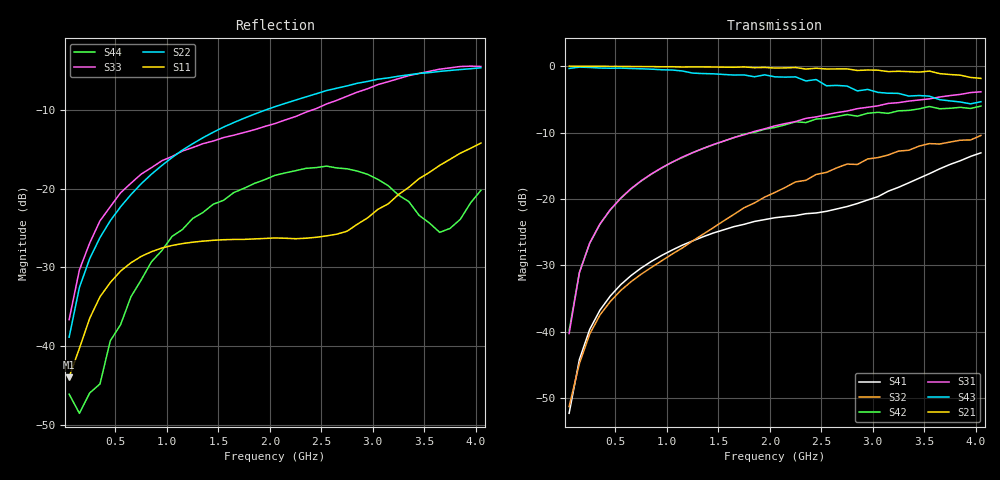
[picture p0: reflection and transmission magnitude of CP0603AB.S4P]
! Network Analyzer HP8720D.07.14 Serial No. US38111185
! 28 Apr 1999  02:06:29
! Frequency 	S11		S21		S31		S41		S12		S22		S23		S24		S13		S23		S33		S34		S14		S24		S34		S44
# HZ  S  DB R 50
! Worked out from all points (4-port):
!   41 points, 50 MHz to 4.05 GHz, reference 50 ohm
!   strongest paths, dB at 50 MHz, 1.05 GHz, 2.05 GHz, 3.05 GHz, 4.05 GHz:
!     S21: 0.0, -0.1, -0.3, -0.6, -1.9
!     S43: -0.4, -0.6, -1.6, -4.0, -5.4
!     S31: -40.2, -14.5, -9.0, -6.0, -3.9
!     S42: -39.8, -14.5, -9.2, -7.0, -6.0
!     S32: -51.2, -28.3, -19.0, -13.8, -10.4
!     S41: -52.2, -27.7, -22.8, -19.6, -13.1
!   lowest |S11| = -43.9 dB at 50 MHz (marker M1), VSWR 1.01, Z = 50.6 - j0.257 ohm
!   |S11| at or under -10 dB: start of sweep to end of sweep
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5e7  -43.93 -23.6  -0.01 -1.1  -41.46 90.6  -52.89 115.5
     -0.02 -0.7  -38.86 41.2  -51.21 84.4  -40.47 85.8
     -40.25 86.7  -51.23 88.0  -36.63 43.5  -0.06 -2.0
     -52.25 97.0  -39.79 80.3  -0.36 -1.7  -46.09 -17.5
1.5e8  -40.27 -64.9  -0.03 -2.4  -31.01 85.8  -44.19 88.0
       -0.03 -2.4  -32.53 55.9  -44.90 88.9  -31.02 85.7
       -31.08 85.5  -44.76 87.7  -30.31 65.5  -0.07 -5.1
       -44.15 87.9  -31.05 85.6  -0.16 -5.0  -48.53 -14.9
2.5e8  -36.46 -80.7  -0.02 -4.0  -26.62 83.1  -39.63 85.8
       -0.04 -4.0  -28.88 59.3  -40.24 86.7  -26.68 82.7
       -26.63 83.2  -40.32 86.8  -26.89 66.4  -0.10 -8.4
       -39.62 85.6  -26.67 82.3  -0.21 -8.3  -45.95 -77.3
9.5e8  -27.53 -129.4  -0.10 -14.9  -15.25 66.3  -28.43 74.9
       -0.11 -15.0  -17.04 36.0  -29.34 86.7  -15.39 64.0
       -15.29 66.3  -29.30 86.5  -16.44 43.8  -0.44 -30.9
       -28.49 74.9  -15.33 63.8  -0.56 -30.8  -27.87 -179.9
2.35e9  -26.28 149.0  -0.39 -36.5  -7.89 30.8  -21.98 58.4
        -0.45 -37.4  -8.32 -29.8  -17.30 77.3  -8.77 30.1
        -7.87 35.1  -17.19 71.5  -10.26 -51.1  -2.02 -75.9
        -22.21 62.6  -8.51 23.9  -2.24 -77.2  -17.40 154.4
3.65e9  -17.02 42.1  -1.34 -59.3  -5.69 -4.7  -15.74 55.5
        -1.14 -57.3  -5.08 -85.9  -10.83 44.9  -6.04 3.5
        -4.66 6.9  -11.73 36.7  -4.80 -117.0  -4.25 -124.2
        -15.46 68.7  -6.43 -7.4  -5.06 -118.6  -25.54 60.6
4.05e9  -14.19 26.5  -1.88 -71.3  -5.56 -17.4  -14.06 40.6
        -1.86 -63.8  -4.62 -107.7  -9.36 31.1  -5.18 -8.0
        -3.87 -3.1  -10.45 26.9  -4.45 -135.1  -5.22 -148.2
        -13.06 58.7  -6.03 -14.6  -5.37 -134.5  -20.19 -12.9
